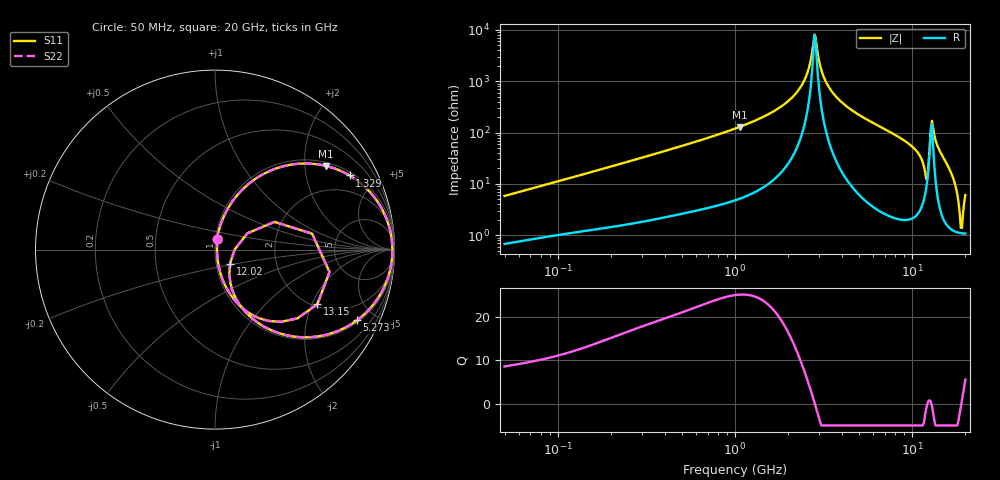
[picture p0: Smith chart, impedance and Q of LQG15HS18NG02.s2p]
!Murata Part Number: LQG15HS18NG02
!These Parameters are Measured in Series Mode Connection
!  o--[Z]--o
!Port1  Port2
!  o-------o
!Freq. Start=50[MHz] Stop=20[GHz], 401[Steps]
# Hz S RI R 50
!Freq.(Hz) S11(Real) S11(Imag) S21(Real) S21(Imag) S12(Real) S12(Imag) S22(Real) S22(Imag)
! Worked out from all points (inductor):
!   401 points, 50 MHz to 20 GHz, reference 50 ohm
!   read as one part in series: L = 18.2 nH near 51.52 MHz
!   highest Q = 25 at 1.062 GHz (marker M1), where L = 19.3 nH
!   self-resonance near 2.811 GHz
!   S11 on the Smith chart (normalised r, x): 50 MHz: 1.01, +0.12; 1.329 GHz: 1.15, +3.54; 5.273 GHz: 1.10, -3.98; 12.02 GHz: 1.17, -0.19; 13.15 GHz: 2.10, -2.20; 20 GHz: 1.02, +0.12
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5e7  0.01 0.0571  0.99 -0.0571  0.99 -0.0571  0.01 0.0571
1.364002e8  0.0332 0.144  0.9668 -0.144  0.9668 -0.144  0.0332 0.144
3.721004e8  0.1538 0.3355  0.8462 -0.3355  0.8462 -0.3355  0.1538 0.3355
1e9  0.5844 0.4732  0.4156 -0.4732  0.4156 -0.4732  0.5844 0.4732
1.061746e9  0.6198 0.4659  0.3802 -0.4659  0.3802 -0.4659  0.6198 0.4659
1.329223e9  0.7497 0.4132  0.2503 -0.4132  0.2503 -0.4132  0.7497 0.4132
2.211938e9  0.9593 0.1615  0.0407 -0.1615  0.0407 -0.1615  0.9593 0.1615
2.531158e9  0.9821 0.074  0.0179 -0.074  0.0179 -0.074  0.9821 0.074
2.728004e9  0.9875 0.0235  0.0125 -0.0235  0.0125 -0.0235  0.9875 0.0235
2.853386e9  0.9883 -0.00712  0.0117 0.00712  0.0117 0.00712  0.9883 -0.00712
3.121702e9  0.9838 -0.0688  0.0162 0.0688  0.0162 0.0688  0.9838 -0.0688
3.572216e9  0.962 -0.1607  0.038 0.1607  0.038 0.1607  0.962 -0.1607
5.273168e9  0.7923 -0.3929  0.2077 0.3929  0.2077 0.3929  0.7923 -0.3929
7.442007e9  0.5193 -0.4884  0.4807 0.4884  0.4807 0.4884  0.5193 -0.4884
1.034674e10  0.198 -0.3755  0.802 0.3755  0.802 0.3755  0.198 -0.3755
1.201863e10  0.0838 -0.0782  0.9162 0.0782  0.9162 0.0782  0.0838 -0.0782
1.257102e10  0.3313 0.1546  0.6687 -0.1546  0.6687 -0.1546  0.3313 0.1546
1.314879e10  0.5704 -0.3044  0.4296 0.3044  0.4296 0.3044  0.5704 -0.3044
1.375312e10  0.2952 -0.3969  0.7048 0.3969  0.7048 0.3969  0.2952 -0.3969
1.670968e10  0.0356 -0.1484  0.9644 0.1484  0.9644 0.1484  0.0356 -0.1484
1.88369e10  0.011 -0.00847  0.989 0.00847  0.989 0.00847  0.011 -0.00847
2e10  0.0142 0.0585  0.9858 -0.0585  0.9858 -0.0585  0.0142 0.0585
